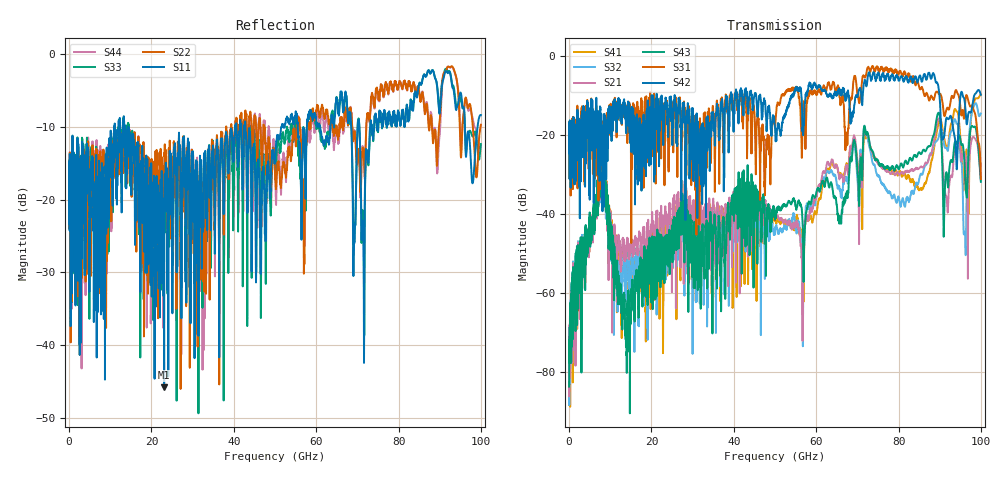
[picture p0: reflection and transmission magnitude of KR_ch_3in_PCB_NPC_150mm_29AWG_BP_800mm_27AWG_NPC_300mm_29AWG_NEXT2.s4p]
# GHz S RI R 45
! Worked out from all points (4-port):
!   4000 points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, 25 MHz to 100 GHz, reference 45 ohm
!   strongest paths, dB at 25 MHz, 25.02 GHz, 50.02 GHz, 75.03 GHz, 100 GHz:
!     S42: -21.3, -17.5, -18.0, -4.3, -9.8
!     S31: -21.2, -13.7, -17.5, -2.9, -31.1
!     S43: -83.8, -45.4, -41.0, -26.4, -31.8
!     S21: -81.7, -47.4, -40.8, -27.2, -27.3
!     S32: -83.4, -45.0, -44.3, -30.5, -14.5
!     S41: -88.4, -51.4, -41.3, -27.1, -9.6
!   lowest |S11| = -45.9 dB at 23.1 GHz (marker M1), VSWR 1.01, Z = 44.7 + j0.331 ohm
!   |S11| at or under -10 dB: start of sweep to 11.02 GHz; 14.38 GHz to 40.34 GHz (25.96 GHz wide, 94.9 % of centre); 42.82 GHz to 51.62 GHz (8.797 GHz wide, 18.6 % of centre)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
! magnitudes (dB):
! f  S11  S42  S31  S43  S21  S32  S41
! 25 MHz  -16.7  -21.3  -21.2  -83.8  -81.7  -83.4  -88.4
! 8.025 GHz  -17.2  -27.6  -24.8  -24.2  -25.2  -25.0  -24.7
! 13.62 GHz  -11.0  -12.9  -12.3  -68.0  -51.7  -61.4  -54.1
! 23.1 GHz  -45.9  -16.9  -19.8  -49.5  -41.9  -47.5  -46.1
! 93.8 GHz  -7.1  -21.7  -8.8  -21.5  -22.9  -16.1  -13.4
! 96.1 GHz  -9.6  -11.7  -13.2  -28.5  -24.6  -44.6  -27.3
! 100 GHz  -8.4  -9.8  -31.1  -31.8  -27.3  -14.5  -9.6
